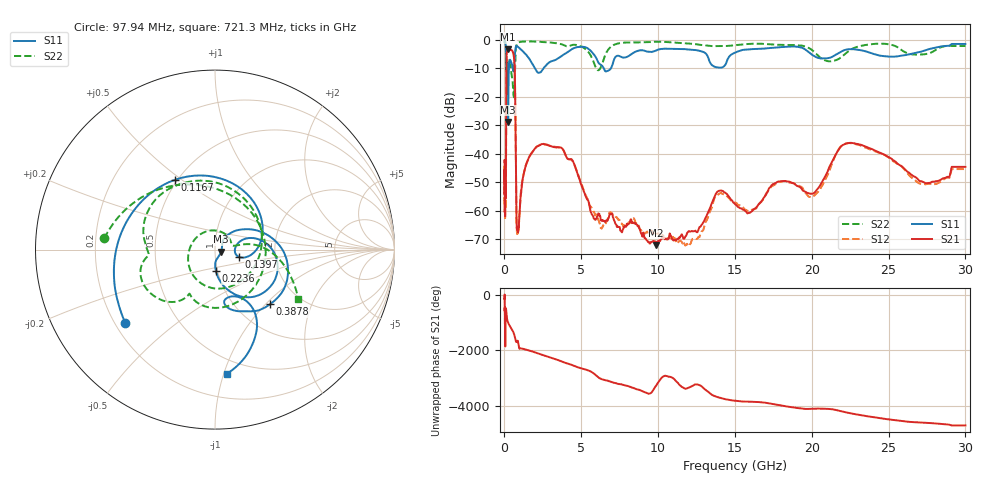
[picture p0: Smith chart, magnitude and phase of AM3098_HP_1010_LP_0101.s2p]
! Date/Time: Thu, Feb 28, 2019 8:42 AM
! Network Analyzer: Agilent Technologies E8364B Rev: A.07.50.67
! Sweep from 0.010 to 30.000 GHz, 1601 Points, Sweep Type: LOG
! Power Supply: 5.022 V, 0.002 A
# Hz S DB R 50
!freq MagS11 AngS11 MagS21 AngS21 MagS12 AngS12 MagS22 AngS22
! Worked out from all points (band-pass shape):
!   1601 points, 10 MHz to 30 GHz, reference 50 ohm
!   highest |S21| = -3.41 dB at 239.9 MHz (marker M1); lowest = -72.0 dB at 9.878 GHz (marker M2)
!   |S21| within 3 dB of the highest: 133 MHz to 623.4 MHz (490.4 MHz wide, 130 % of centre)
!   lowest |S11| = -28.9 dB at 238.7 MHz (marker M3), VSWR 1.07, Z = 53.5 - j1.19 ohm
!   |S11| at or under -10 dB: 199.9 MHz to 289.9 MHz (90.01 MHz wide, 36.8 % of centre); 1.975 GHz to 2.553 GHz (577.6 MHz wide, 25.5 % of centre); 6.456 GHz to 6.939 GHz (483 MHz wide, 7.21 % of centre)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
!   |S22| runs from -20.3 to -0.5 dB; largest |S21 - S12| = 0.013
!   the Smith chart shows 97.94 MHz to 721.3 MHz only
!   S11 on the Smith chart (normalised r, x): 97.94 MHz: 0.24, -0.34; 116.7 MHz: 0.48, +0.47; 139.7 MHz: 1.30, -0.11; 223.6 MHz: 0.98, -0.24; 387.8 MHz: 1.42, -1.06; 721.3 MHz: 0.39, -1.03
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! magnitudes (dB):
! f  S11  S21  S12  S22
! 10 MHz  -0.3  -43.0  -44.4  -0.5
! 38.04 MHz  -0.5  -58.9  -60.6  -0.8
! 97.94 MHz  -3.8  -46.9  -50.1  -4.2
! 116.7 MHz  -7.0  -17.9  -17.9  -10.9
! 139.7 MHz  -17.1  -5.2  -5.2  -10.9
! 144.7 MHz  -19.1  -4.8  -4.8  -10.8
! 223.6 MHz  -18.5  -3.5  -3.5  -8.5
! 238.7 MHz  -28.9  -3.4  -3.4  -8.7
! 239.9 MHz  -28.9  -3.4  -3.4  -8.6
! 387.8 MHz  -7.3  -3.7  -3.6  -8.9
! 550.5 MHz  -10.5  -4.4  -4.4  -16.7
! 659.1 MHz  -6.8  -9.6  -9.6  -15.6
! 721.3 MHz  -3.2  -30.8  -30.9  -5.3
! 781.4 MHz  -2.3  -62.0  -63.1  -2.0
! 842.3 MHz  -2.4  -66.6  -67.4  -1.3
! 2.084 GHz  -11.1  -37.6  -37.6  -0.7
! 3.742 GHz  -5.7  -38.1  -38.2  -1.7
! 7.926 GHz  -6.2  -65.6  -65.1  -1.0
! 9.878 GHz  -3.8  -72.0  -68.1  -0.8
! 20.1 GHz  -5.6  -54.0  -54.9  -4.1
! 22.56 GHz  -3.4  -36.2  -36.4  -3.5
! 30 GHz  -1.6  -44.6  -45.4  -2.3
